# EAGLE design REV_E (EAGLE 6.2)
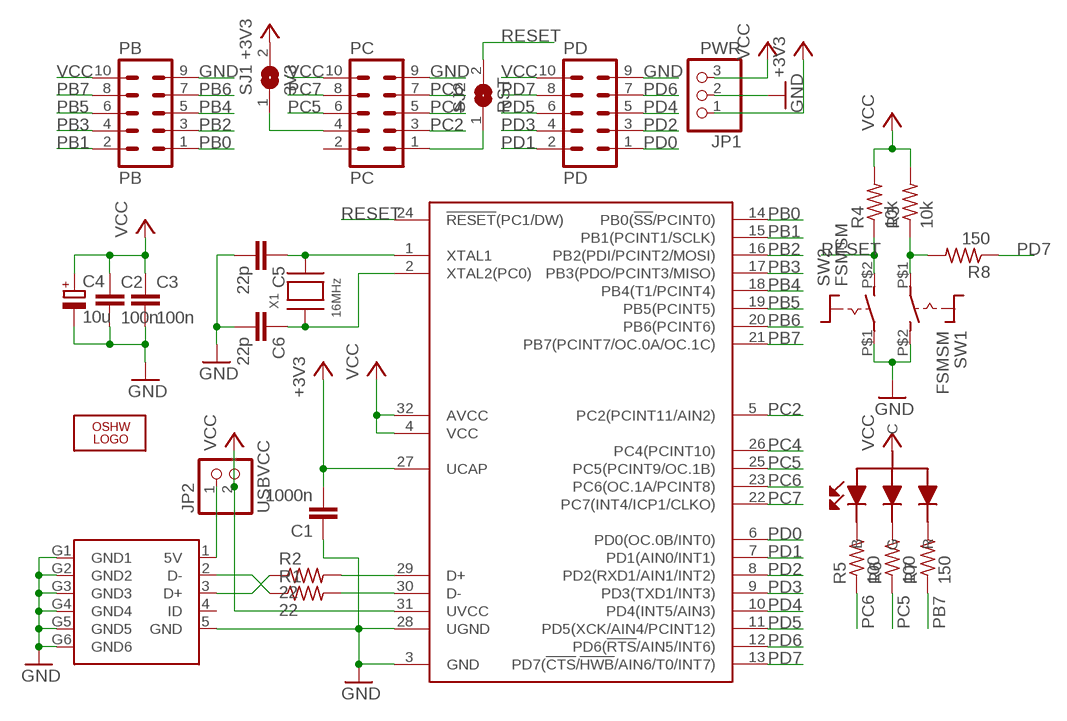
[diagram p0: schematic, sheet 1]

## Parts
C1  1000n  C-EUC0805  [C0805]
C2  100n  C-EUC0805  [C0805]
C3  100n  C-EUC0805  [C0805]
C4  10u  CPOL-EUSMCA  [SMC_A]
C5  22p  C-EUC0805  [C0805]
C6  22p  C-EUC0805  [C0805]
JP1  PWR  PINHD-1X3  [1X03]
JP2  USBVCC  PINHD-1X2  [1X02]
LED1  CLVBA-FKA  [PLCC4]
LOGO1  OSHW_LOGO_10MIL  [OSHW_10X500_NOTEXT_MASK]
PB  PB  ML10  [ML10]
PC  PC  ML10  [ML10]
PD  PD  ML10  [ML10]
R1  22  R-US_R0805  [R0805]
R2  22  R-US_R0805  [R0805]
R3  10k  R-US_R0805  [R0805]
R4  10k  R-US_R0805  [R0805]
R5  100  R-US_R0805  [R0805]
R6  100  R-US_R0805  [R0805]
R7  150  R-US_R0805  [R0805]
R8  150  R-US_R0805  [R0805]
SJ1  3V3  SJ  [SJ]
SJ2  RST  SJ  [SJ]
SW1  FSMSM  [FSMSM]
SW2  FSMSM  [FSMSM]
U1  AT90USB162  [VQFP32]
X1  16MHz  XTALNX5032  [NX5032]
X2  10118193  [10118193]

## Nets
+3V3: C1.2 JP1.1 SJ1.2 U1.27(UCAP)
GND: C1.1 C2.2 C3.2 C4.- C5.2 C6.2 JP1.2 PB.9 PC.9 PD.9 SW1.P$2(S) SW2.P$1(P) U1.3(GND) U1.28(UGND) X2.5(GND) X2.G1(GND1) X2.G2(GND2) X2.G3(GND3) X2.G4(GND4) X2.G5(GND5) X2.G6(GND6)
LED_B: LED1.3(B) R5.2
LED_G: LED1.4(G) R6.2
LED_R: LED1.1(R) R7.2
N$1: R1.2 U1.30(D-)
N$2: R2.1 X2.3(D+)
N$3: R1.1 X2.2(D-)
N$4: R2.2 U1.29(D+)
N$9: PC.4 SJ1.1
N$10: JP2.1 X2.1(5V)
N$12: C6.1 U1.2(XTAL2(PC0)) X1.P$1
N$13: C5.1 U1.1(XTAL1) X1.P$2
N$14: PC.1 SJ2.1
N$16: R3.1 R8.2 SW1.P$1(P)
PB0: PB.1 U1.14(PB0(!SS!/PCINT0))
PB1: PB.2 U1.15(PB1(PCINT1/SCLK))
PB2: PB.3 U1.16(PB2(PDI/PCINT2/MOSI))
PB3: PB.4 U1.17(PB3(PDO/PCINT3/MISO))
PB4: PB.5 U1.18(PB4(T1/PCINT4))
PB5: PB.6 U1.19(PB5(PCINT5))
PB6: PB.7 U1.20(PB6(PCINT6))
PB7: PB.8 R7.1 U1.21(PB7(PCINT7/OC.0A/OC.1C))
PC2: PC.3 U1.5(PC2(PCINT11/AIN2))
PC4: PC.5 U1.26(PC4(PCINT10))
PC5: PC.6 R6.1 U1.25(PC5(PCINT9/OC.1B))
PC6: PC.7 R5.1 U1.23(PC6(OC.1A/PCINT8))
PC7: PC.8 U1.22(PC7(INT4/ICP1/CLKO))
PD0: PD.1 U1.6(PD0(OC.0B/INT0))
PD1: PD.2 U1.7(PD1(AIN0/INT1))
PD2: PD.3 U1.8(PD2(RXD1/AIN1/INT2))
PD3: PD.4 U1.9(PD3(TXD1/INT3))
PD4: PD.5 U1.10(PD4(INT5/AIN3))
PD5: PD.6 U1.11(PD5(XCK/AIN4/PCINT12))
PD6: PD.7 U1.12(PD6(!RTS!/AIN5/INT6))
PD7: PD.8 R8.1 U1.13(PD7(!CTS!/!HWB!/AIN6/T0/INT7))
RESET: R4.1 SJ2.2 SW2.P$2(S) U1.24(!RESET!(PC1/DW))
VCC: C2.1 C3.1 C4.+ JP1.3 JP2.2 LED1.2(C) PB.10 PC.10 PD.10 R3.2 R4.2 U1.4(VCC) U1.31(UVCC) U1.32(AVCC)
Unconnected: PC.2 X2.4(ID)

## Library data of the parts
C1-C3 C5 C6 = rcl:C-EU: CAPACITOR, European symbol
C4 = rcl:CPOL-EU: POLARIZED CAPACITOR, European symbol
JP1 = pinhead:PINHD-1X3: PIN HEADER
JP2 = pinhead:PINHD-1X2: PIN HEADER
LED1 = led-cree:CLVBA-FKA
LOGO1 = ohw-logo:OSHW_LOGO_10MIL
PB PC PD = con-harting-ml2:ML10: HARTING; OC_FARNELL: unknown; OC_NEWARK: unknown
R1-R8 = adafruit:R-US_: RESISTOR, American symbol
SJ1 SJ2 = jumper:SJ: SMD solder JUMPER
SW1 SW2 = switch:FSMSM
U1 = at90usb:AT90USB162
X1 = adafruit:XTAL: Low cost SMT crystals, no capacitors included
X2 = con-fci:10118193

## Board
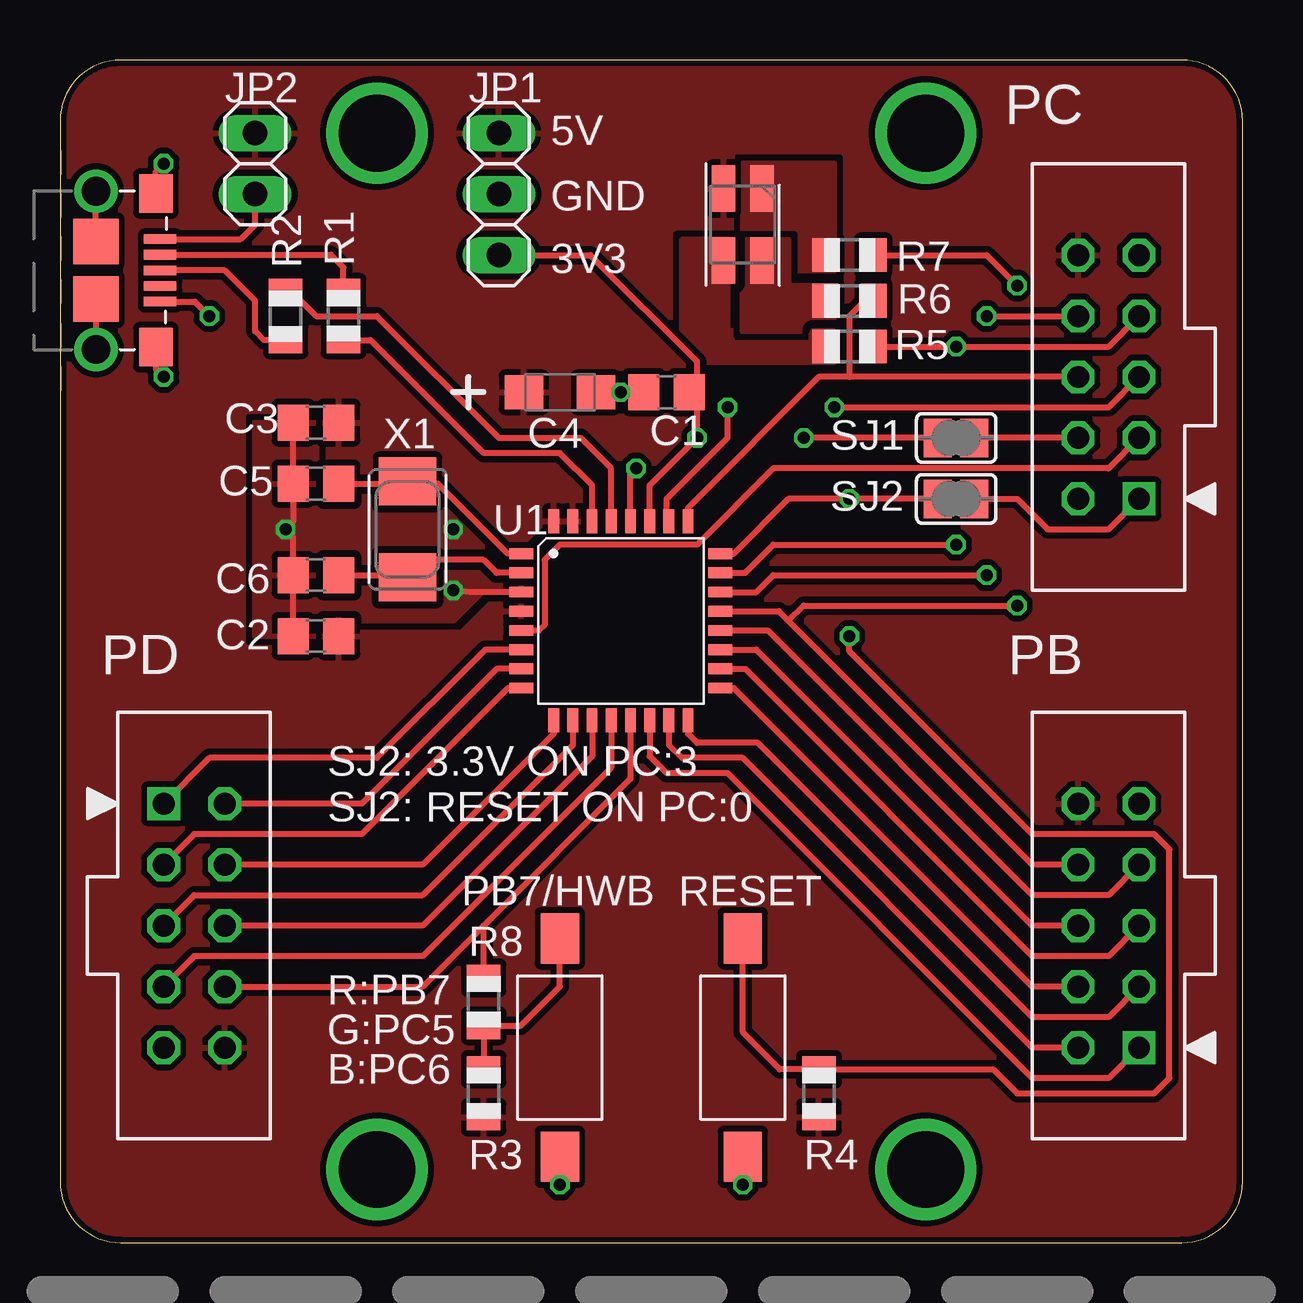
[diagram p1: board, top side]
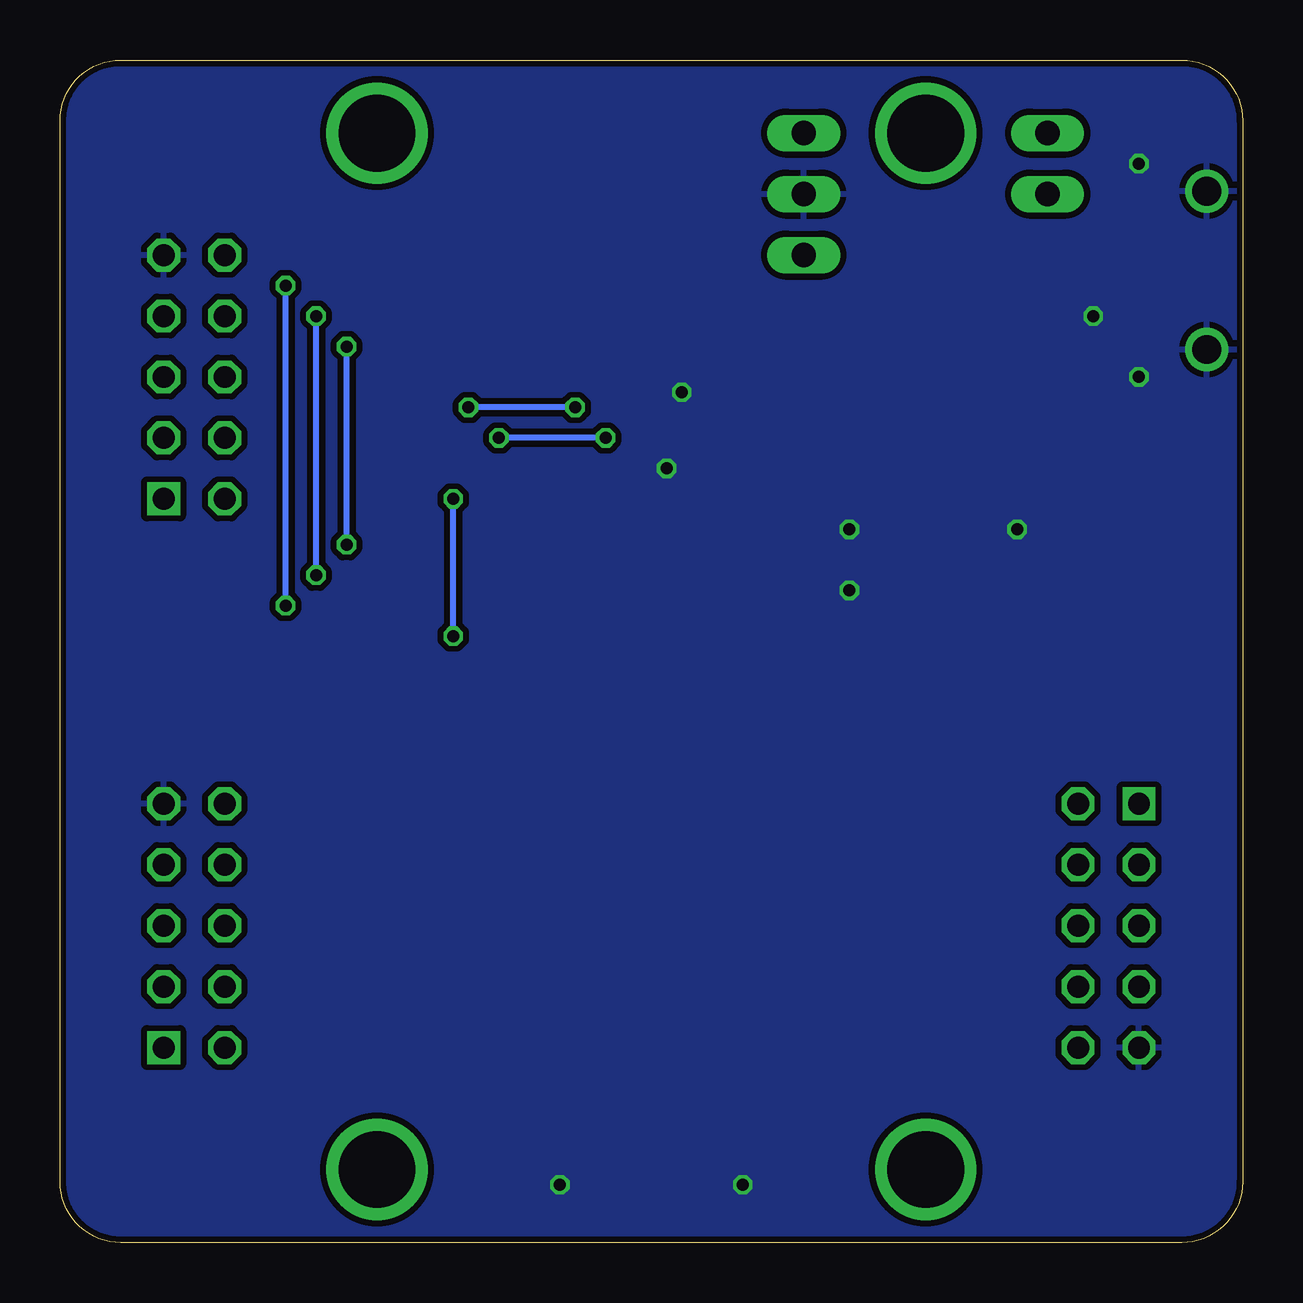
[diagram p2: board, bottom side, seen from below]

Size 49.28 x 49.28 mm. Coordinates in mm from the lower left corner, seen from the top.
Outline: 49.28,2.54 49.28,46.74 arc90 46.74,49.28 2.54,49.28 arc90 0,46.74 0,2.54 arc90 2.54,0 46.74,0 arc90 49.28,2.54
Copper layers (1*2*15*16): Top 0.035mm / dielectric 0.2mm / layer 2 0.0175mm / dielectric 1.1mm / layer 15 0.0175mm / dielectric 0.2mm / Bottom 0.035mm
Design rules: minimum track width 6mil, minimum drill 12mil, track to track 6mil, track to pad 6mil, pad to pad 6mil, via to via 6mil, smd to smd 0mil, copper to edge 10mil, drill to drill 10mil, minimum pad ring 6mil, minimum via ring 6mil, stop-mask expansion 2mil, vias tented up to drill 25mil, thermal gap 10mil

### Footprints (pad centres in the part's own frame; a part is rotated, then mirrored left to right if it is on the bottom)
C0805 = smd 1.3 x 1.5: 1 -0.95,0; 2 0.95,0
SMC_A = smd 1.6 x 1.4: + -1.5,0; - 1.5,0
1X03 = drill 1.016 long: 1 -2.54,0; 2 0,0; 3 2.54,0
1X02 = drill 1.016 long: 1 -1.27,0; 2 1.27,0
PLCC4 = smd 1.93 x 0.965: 1 -1.5,0.8; 2 -1.5,-0.8; 3 1.5,-0.8; 4 1.5,0.8
ML10 = drill 0.914 square: 1 -5.08,-1.27 | drill 0.914 octagon: 2 -5.08,1.27; 3 -2.54,-1.27; 4 -2.54,1.27; 5 0,-1.27; 6 0,1.27; 7 2.54,-1.27; 8 2.54,1.27; 9 5.08,-1.27; 10 5.08,1.27
R0805 = smd 1.1 x 1.4: 1 -1,0; 2 1,0
SJ = smd 1.168 x 1.6: 1 -0.762,0; 2 0.762,0
FSMSM = smd 2.1 x 1.6: P$1 -4.55,0; P$2 4.55,0
VQFP32 = smd 1 x 0.45: 1 -4.15,2.8; 2 -4.15,2; 3 -4.15,1.2; 4 -4.15,0.4; 5 -4.15,-0.4; 6 -4.15,-1.2; 7 -4.15,-2; 8 -4.15,-2.8; 17 4.15,-2.8; 18 4.15,-2; 19 4.15,-1.2; 20 4.15,-0.4; 21 4.15,0.4; 22 4.15,1.2; 23 4.15,2; 24 4.15,2.8 | smd 0.45 x 1: 9 -2.8,-4.15; 10 -2,-4.15; 11 -1.2,-4.15; 12 -0.4,-4.15; 13 0.4,-4.15; 14 1.2,-4.15; 15 2,-4.15; 16 2.8,-4.15; 25 2.8,4.15; 26 2,4.15; 27 1.2,4.15; 28 0.4,4.15; 29 -0.4,4.15; 30 -1.2,4.15; 31 -2,4.15; 32 -2.8,4.15
NX5032 = smd 2 x 2.4: P$1 2,0; P$2 -2,0
10118193 = smd 0.4 x 1.35: 1 -1.3,2.775; 2 -0.65,2.775; 3 0,2.775; 4 0.65,2.775; 5 1.3,2.775 | smd 1.6 x 1.4: G1 -3.2,2.6; G2 3.2,2.6 | smd 1.9 x 1.9: G3 -1.2,0.1; G4 1.2,0.1 | drill 1.2 pad 1.6: G5 -3.3,0.1; G6 3.3,0.1

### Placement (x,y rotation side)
C1  25.27,35.43 0 top
C2  10.67,25.27 180 top
C3  10.67,34.16 180 top
C4  20.83,35.43 0 top
C5  10.67,31.62 180 top
C6  10.67,27.81 180 top
JP1  18.29,43.69 90 top
JP2  8.13,44.96 90 top
LED1  28.45,42.42 270 top
LOGO1  31.62,11.3 0 bottom
PB  43.69,13.21 90 top
PC  43.69,36.07 90 top
PD  5.59,13.21 270 top
R1  11.81,38.61 270 top
R2  9.4,38.61 90 top
R3  17.65,6.22 270 top
R4  31.62,6.22 270 top
R5  32.89,37.34 180 top
R6  32.89,39.24 180 top
R7  32.89,41.15 180 top
R8  17.65,10.03 270 top
SJ1  37.34,33.53 180 top
SJ2  37.34,30.99 180 top
SW1  20.83,8.13 270 top
SW2  28.45,8.13 90 top
U1  23.37,25.91 0 top
X1  14.48,29.72 270 top
X2  1.4,40.51 270 top

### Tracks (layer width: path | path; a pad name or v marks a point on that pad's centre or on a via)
+3V3  (via drill 0.5, 0.5 pad 0.25)
  Top 0.254: U1.27 24.57,31.55 v26.54,33.53 26.54,35.43 | SJ1.2 v30.99,33.53 | JP1.1 22.1,41.15 26.54,36.7 26.54,35.43 | C1.2 26.54,35.43
  Bottom 0.254: v26.54,33.53 v30.99,33.53
GND  (via drill 0.5, 0.5 pad 0.25)
  Top 0.254: U1.28 23.77,32.02 v24,32.26 | C2.2 C6.2 9.72,29.4 v9.4,29.72 9.72,30.04 C5.2 C3.2 | X2.5 5.62,39.21 v6.22,38.61 | X2.G3 X2.G5 | X2.G4 X2.G6 | v20.83,2.41 SW1.P$2 | v28.45,2.41 SW2.P$1 | C4.- v23.37,35.43 C1.1 | U1.3 17.09,27.11 v16.38,27.18 | X2.G2 4,36.39 v4.32,36.07 | X2.G1 4,44.64 v4.32,44.96
  other vias: 16.38,29.72
  pour Bottom (isolate 0.254): -0.76,-0.76 50.04,-0.76 50.04,50.04 -0.76,50.04
  pour Top (isolate 0.305): 19.56,27.18 17.65,27.18 16.38,25.91 10.67,25.91 10.67,25.27 8.13,25.27 8.13,34.16 10.67,34.16 10.67,31.62 15.11,31.62
LED_B
  pour Top (isolate 0.254, rank 2, no thermals): 27.81,41.78 25.91,41.78 25.91,37.34 26.54,36.7 32.26,36.7 32.26,37.97 27.81,37.97
LED_G
  pour Top (isolate 0.406, no thermals): 28.45,41.78 30.35,41.78 30.35,39.88 32.26,39.88 32.26,37.97 28.45,37.97
LED_R
  pour Top (isolate 0.254, rank 2, no thermals): 28.45,40.51 32.26,40.51 32.26,44.96 28.45,44.96
N$1
  Top 0.254: U1.30 22.17,31.55 20.83,32.89 17.65,32.89 12.94,37.61 R1.2
N$2
  Top 0.254: R2.1 8.49,37.61 8.13,37.97 8.13,39.24 6.86,40.51 X2.3
N$3
  Top 0.254: X2.2 11.29,41.16 11.81,40.64 R1.1
N$4
  Top 0.254: U1.29 22.97,32.26 21.7,33.53 18.29,33.53 13.21,38.61 10.67,38.61 9.67,39.61 R2.2
N$5
  cutout Top: 19.56,29.08 19.56,22.73 20.19,22.1 26.54,22.1 27.18,22.73 27.18,29.08 26.54,29.72 20.19,29.72
N$6  (via drill 3.2)
  other vias: 13.21,3.05
N$8  (via drill 3.2)
  other vias: 36.07,3.05
N$9
  Top 0.254: PC.4 SJ1.1
N$10
  Top 0.254: X2.1 7.52,41.81 8.13,42.42 JP2.1
N$11  (via drill 3.2)
  other vias: 13.21,46.23
N$12
  Top 0.254: U1.2 18.19,27.91 17.65,28.45 15.21,28.45 X1.P$1 14.38,27.81 C6.1
N$13
  Top 0.254: U1.1 18.66,28.71 15.75,31.62 14.57,31.62 X1.P$2 14.38,31.62 C5.1
N$14
  Top 0.254: SJ2.1 39.88,30.99 41.15,29.72 43.69,29.72 PC.1
N$15  (via drill 3.2)
  other vias: 36.07,46.23
N$16
  Top 0.254: R3.1 R8.2 19.19,9.03 20.83,10.67 SW1.P$1
PB0
  Top 0.254: U1.14 24.57,20.26 25.27,19.56 27.81,19.56 40.51,6.86 43.69,6.86 PB.1
PB1
  Top 0.254: U1.15 25.37,20.73 25.91,20.19 28.45,20.19 40.51,8.13 PB.2
PB2
  Top 0.254: U1.16 26.17,21.2 26.54,20.83 29.08,20.83 40.51,9.4 43.69,9.4 PB.3
PB3
  Top 0.254: U1.17 28.07,23.11 40.51,10.67 PB.4
PB4
  Top 0.254: U1.18 28.54,23.91 40.51,11.94 43.69,11.94 PB.5
PB5
  Top 0.254: U1.19 29.01,24.71 40.51,13.21 PB.6
PB6
  Top 0.254: U1.20 29.48,25.51 40.51,14.48 43.69,14.48 PB.7
PB7  (via drill 0.5 pad 0.25)
  Top 0.254: U1.21 29.95,26.31 30.35,25.91 | PB.8 40.51,15.75 30.35,25.91 | 30.35,25.91 30.99,26.54 v39.88,26.54 | R7.1 38.61,41.15 v39.88,39.88
  Bottom 0.254: v39.88,26.54 v39.88,39.88
PC2
  Top 0.254: U1.5 19.96,25.51 20.19,25.74 20.19,28.45 20.83,29.08 26.54,29.08 29.72,32.26 43.69,32.26 PC.3
PC4  (via drill 0.5 pad 0.25)
  Top 0.254: U1.26 25.37,30.26 25.27,30.35 25.27,30.99 27.81,33.53 v27.81,34.8 | v32.26,34.8 43.69,34.8 PC.5
  Bottom 0.254: v27.81,34.8 v32.26,34.8
PC5
  Top 0.254: U1.25 26.17,30.61 31.62,36.07 32.89,36.07 | PC.6 32.89,36.07 | R6.1 33.53,39.24 32.89,38.61 32.89,36.07
PC6  (via drill 0.5 pad 0.25)
  Top 0.254: U1.23 28.54,27.91 29.72,29.08 v37.34,29.08 | PC.7 43.69,37.34 v37.34,37.34 R5.1
  Bottom 0.254: v37.34,29.08 v37.34,37.34
PC7  (via drill 0.5 pad 0.25)
  Top 0.254: U1.22 29.01,27.11 29.72,27.81 v38.61,27.81 | v38.61,38.61 PC.8
  Bottom 0.254: v38.61,27.81 v38.61,38.61
PD0
  Top 0.254: U1.6 17.72,24.71 13.21,20.19 6.22,20.19 PD.1
PD1
  Top 0.254: U1.7 18.19,23.91 12.57,18.29 PD.2
PD2
  Top 0.254: U1.8 18.66,23.11 12.57,17.02 5.59,17.02 PD.3
PD3
  Top 0.254: U1.9 20.57,21.2 15.11,15.75 PD.4
PD4
  Top 0.254: U1.10 21.37,20.73 15.11,14.48 5.59,14.48 PD.5
PD5
  Top 0.254: U1.11 22.17,20.26 15.11,13.21 PD.6
PD6
  Top 0.254: U1.12 22.97,19.79 15.11,11.94 5.59,11.94 PD.7
PD7
  Top 0.254: U1.13 23.77,19.32 17.65,13.21 | PD.8 15.11,10.67 17.65,13.21 | R8.1 17.65,13.21
RESET  (via drill 0.5 pad 0.25)
  Top 0.254: U1.24 28.07,28.71 30.35,30.99 v32.89,30.99 SJ2.2 | v32.89,25.27 32.89,24.64 40.51,17.02 45.59,17.02 46.23,16.38 46.23,6.86 45.59,6.22 39.88,6.22 38.88,7.22 R4.1 29.99,7.22 28.45,8.76 SW2.P$2 28.55,12.57
  Bottom 0.254: v32.89,25.27 v32.89,30.99
VCC
  pour Top (isolate 0.254, rank 5): -0.76,50.04 50.04,50.04 50.04,-0.76 -0.76,-0.76

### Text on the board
tNames: 5V | GND | 3V3 | SJ2: 3.3V ON PC:3 | SJ2: RESET ON PC:0 | PB7/HWB | RESET | R:PB7 | G:PC5 | B:PC6
tValues: 1 | 1 | 1 | 1
tStop: 2013
bStop: slashhome.se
